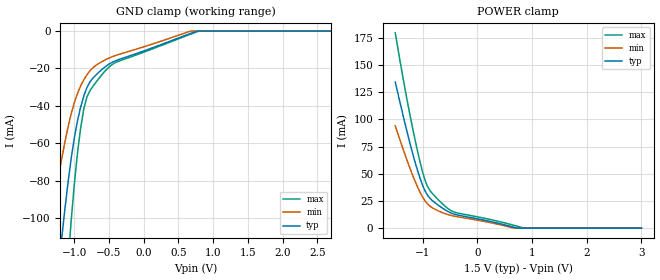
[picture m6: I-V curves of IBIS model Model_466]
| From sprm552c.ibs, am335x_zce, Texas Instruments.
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| Model based on original model for BCSHTLTCSCDVPBFZ_SSDHV
|   Sub model VREF_HALFTERM_11MA_10PER_1P5
[model]   Model_466
|[Description]  [1.5V-INPUT-HALFTERM:11MA-X, IND, 10%]
|   Half Thevenin termination (Rth = 100R whith RExt = 50R)
|   (ODT[1:0] = "11") VRef mode, 0.73 * RExt = 1.325 * Iout (I[2:0]
|   = "110"), 11mA nominal with Rext = 50R,Industrial temperature
|   range (-40C to 125C, 25C nominal),10% power supply tolerance
|[Input Load]   HALFTERM:11MA
|[Output Drive]
|Voltage   1.5V
|Mode   INPUT
Model_type   Input
Polarity   Non-Inverting
Vinl =  0.65
Vinh =  0.85
C_comp   1.865048p   1.676829p   1.989968p
[Model Spec]
Vinl   0.65   0.575   0.725
Vinh   0.85   0.775   0.925
[Temperature Range]   25   125   -40
[Voltage Range]   1.5   1.35   1.65
[POWER_clamp]
-1.5V     134.4mA    94mA       179.5mA
-1.364V   105mA      73.71mA    139.7mA
-1.227V   77.25mA    54.59mA    103.1mA
-1.091V   52.71mA    37.66mA    70.29mA
-1V       39.42mA    28.56mA    51.52mA
-954.5mV  34.19mA    25.02mA    43.93mA
-863.6mV  27.33mA    20.17mA    34.44mA
-545.5mV  15.53mA    12.63mA    18.34mA
-363.6mV  12.09mA    10.51mA    13.95mA
681.8mV   684.6uA    0A         2.461mA
863.6mV   0A         0A         0A
3V        0A         0A         0A
[GND_clamp]
-1.5V     -232.3mA   -140.9mA   -378.1mA
-1.364V   -178.4mA   -108.4mA   -289.4mA
-1.182V   -110.9mA   -68.38mA   -175.7mA
-1.091V   -81.03mA   -51.39mA   -124mA
-1.045V   -68.17mA   -44.25mA   -101.4mA
-954.5mV  -48.05mA   -33.32mA   -65.28mA
-863.6mV  -34.73mA   -26.07mA   -41.6mA
-772.7mV  -27.05mA   -21.15mA   -31.78mA
-636.4mV  -21.64mA   -17.09mA   -24.88mA
-409.1mV  -15.93mA   -13.09mA   -16.87mA
772.7mV   0A         0A         -245.3uA
3V        0A         0A         0A
